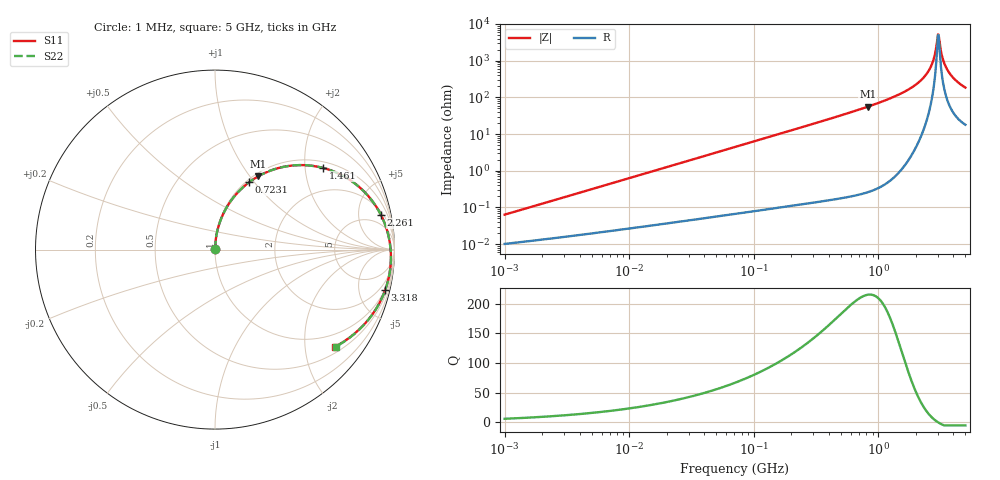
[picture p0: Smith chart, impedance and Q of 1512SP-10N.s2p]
!AWR Design Environment (3650) Fri Sep 11 12:29:03 2020
!freq-unit  param-type  data-format  keyword  impedance-ohms
# MHz  S  MA  R  50
!Freq  MagS11  AngS11  MagS21  AngS21  MagS12  AngS12  MagS22  AngS22
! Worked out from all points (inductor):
!   801 points, 1 MHz to 5 GHz, reference 50 ohm
!   read as one part in series: L = 9.98 nH near 1.044 MHz
!   highest Q = 215 at 821.7 MHz (marker M1), where L = 10.8 nH
!   self-resonance near 3.014 GHz
!   S11 on the Smith chart (normalised r, x): 1 MHz: 1.00, +0.00; 723.1 MHz: 1.03, +0.94; 1.461 GHz: 1.18, +2.50; 2.261 GHz: 2.49, +8.93; 3.318 GHz: 0.93, -8.36; 5 GHz: 0.64, -2.70
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1  0.0006144 80.5  0.9999 -0.0  0.9999 -0.0  0.0006144 80.5
4.168304  0.002532 85.8  0.9998 -0.2  0.9998 -0.2  0.002532 85.8
17.19065  0.01042 87.5  0.9996 -0.6  0.9996 -0.6  0.01042 87.5
70.89654  0.04293 86.5  0.9984 -2.6  0.9984 -2.6  0.04293 86.5
295.5183  0.1778 78.6  0.9828 -10.9  0.9828 -10.9  0.1778 78.6
723.1289  0.4215 63.1  0.9048 -26.6  0.9048 -26.6  0.4214 63.1
821.7401  0.4737 59.5  0.8784 -30.2  0.8784 -30.2  0.4736 59.5
1218.757  0.6619 45.3  0.7459 -44.3  0.7459 -44.3  0.6617 45.3
1460.726  0.756 37.0  0.649 -52.6  0.649 -52.6  0.7558 37.0
1866.293  0.8745 23.7  0.4722 -65.5  0.4722 -65.5  0.8743 23.7
2260.778  0.9442 11.9  0.2985 -76.2  0.2985 -76.2  0.9441 11.9
2461.9  0.9648 6.3  0.2141 -80.4  0.2141 -80.4  0.9646 6.3
2652.506  0.9764 1.4  0.1382 -82.7  0.1382 -82.7  0.9763 1.4
2797.623  0.9809 -2.1  0.08395 -81.4  0.08395 -81.4  0.9809 -2.1
2950.679  0.9823 -5.7  0.0325 -63.6  0.0325 -63.6  0.9823 -5.7
3014.221  0.9819 -7.1  0.01885 -24.6  0.01885 -24.6  0.982 -7.1
3112.109  0.9805 -9.2  0.03302 45.5  0.03302 45.5  0.9806 -9.2
3317.525  0.9743 -13.5  0.09351 63.3  0.09351 63.3  0.9745 -13.5
3536.499  0.9641 -17.7  0.1549 63.5  0.1549 63.5  0.9645 -17.7
3851.111  0.9451 -23.1  0.2332 60.1  0.2332 60.1  0.9456 -23.1
4329.904  0.9109 -30.4  0.3312 53.9  0.3312 53.9  0.9117 -30.4
5000  0.8613 -38.9  0.4338 45.9  0.4338 45.9  0.8627 -38.9
